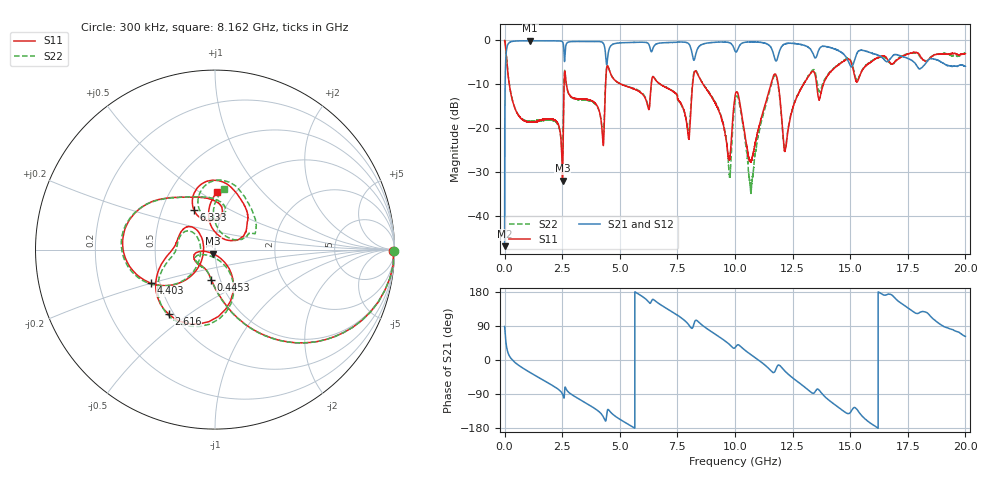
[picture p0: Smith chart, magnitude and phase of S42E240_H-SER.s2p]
!{S42E240}
!Johanson Technology Inc.
!www.johansontechnology.com
!Test Board Conditions:
!Substrate Type  RO4350B
!Substrate Thickness  50 mil
!Substrate Dk  3.66
!TL Type: GCPW
!TL Trace Width  60 mil
!TL Gap  10 mil
!Electrode orientation  Horizontal
!DUT TOPOLOGY	SERIES
!Mounting Pad LxW  14x55 mil
! Created Wed Nov 25 22:07:07 2020
# khz S ma R 50
! 2 Port Network Data from SP1.SP block
! freq  magS11  angS11  magS21  angS21  magS12  angS12  magS22  angS22
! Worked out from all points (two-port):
!   20001 points, 300 kHz to 20 GHz, reference 50 ohm
!   highest |S21| = -0.07 dB at 1.105 GHz (marker M1); lowest = -46.9 dB at 300 kHz (marker M2)
!   |S21| within 3 dB of the highest: 4.493 GHz to 8.139 GHz (3.646 GHz wide, 57.7 % of centre); 8.301 GHz to 11.67 GHz (3.369 GHz wide, 33.7 % of centre)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
!   lowest |S11| = -32.0 dB at 2.513 GHz (marker M3), VSWR 1.05, Z = 48.9 - j2.23 ohm
!   |S11| at or under -10 dB: 203.5 MHz to 2.583 GHz (2.379 GHz wide, 171 % of centre); 2.68 GHz to 4.383 GHz (1.703 GHz wide, 48.2 % of centre); 8.618 GHz to 11.56 GHz (2.942 GHz wide, 29.2 % of centre)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
!   |S22| runs from -34.9 to 0.0 dB; largest |S21 - S12| = 0.017
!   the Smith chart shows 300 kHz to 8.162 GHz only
!   S11 on the Smith chart (normalised r, x): 300 kHz: open; 445.3 MHz: 0.91, -0.31; 2.616 GHz: 0.47, -0.42; 4.403 GHz: 0.45, -0.20; 6.333 GHz: 0.72, +0.34; 8.162 GHz: 0.83, +0.60
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300  0.994 -0.3  0.004503 88.7  0.004542 89.0  0.9953 -0.5
116300  0.4958 -64.3  0.8662 25.6  0.867 25.6  0.4974 -64.4
445300  0.1687 -97.0  0.9832 -6.3  0.9841 -6.3  0.17 -96.7
1105300  0.117 -125.3  0.9917 -33.0  0.9896 -33.0  0.1196 -122.1
2513300  0.0252 -115.5  0.9646 -89.5  0.9647 -89.5  0.04355 -99.6
2616300  0.4431 -125.6  0.6551 -73.1  0.6548 -73.1  0.4517 -123.5
3334300  0.2143 158.2  0.9736 -106.8  0.9732 -106.8  0.2105 167.9
4240300  0.08734 142.7  0.9535 -145.6  0.9536 -145.6  0.09418 155.5
4403300  0.4013 -152.1  0.59 -158.0  0.5903 -158.0  0.4126 -152.7
6333300  0.2519 118.0  0.7806 150.2  0.7799 150.1  0.2543 111.2
6667300  0.3288 67.0  0.9264 150.0  0.9246 150.0  0.3306 58.9
7965300  0.08404 39.9  0.9291 94.9  0.9276 95.1  0.09751 47.1
8162300  0.3232 87.5  0.6525 85.2  0.6506 85.1  0.3429 80.5
9212300  0.1772 -25.8  0.9544 65.1  0.9572 65.2  0.1799 -21.3
9754300  0.04383 15.6  0.9432 41.2  0.9446 41.3  0.0297 -4.7
1.00003e7  0.2309 37.1  0.7578 32.2  0.7569 32.3  0.2006 38.0
1.06943e7  0.04102 24.0  0.9616 14.0  0.9621 14.0  0.01883 -171.7
1.16763e7  0.3972 23.2  0.6927 -33.2  0.6907 -33.1  0.3805 18.4
1.21783e7  0.05576 7.3  0.9156 -29.9  0.9176 -30.0  0.05925 -4.7
1.33343e7  0.4364 -3.8  0.7541 -86.7  0.757 -86.6  0.4517 -15.7
1.66673e7  0.5787 -110.5  0.5923 174.1  0.5798 174.1  0.5697 -122.0
2e7  0.7074 161.9  0.5052 62.2  0.5045 63.2  0.7111 148.1
